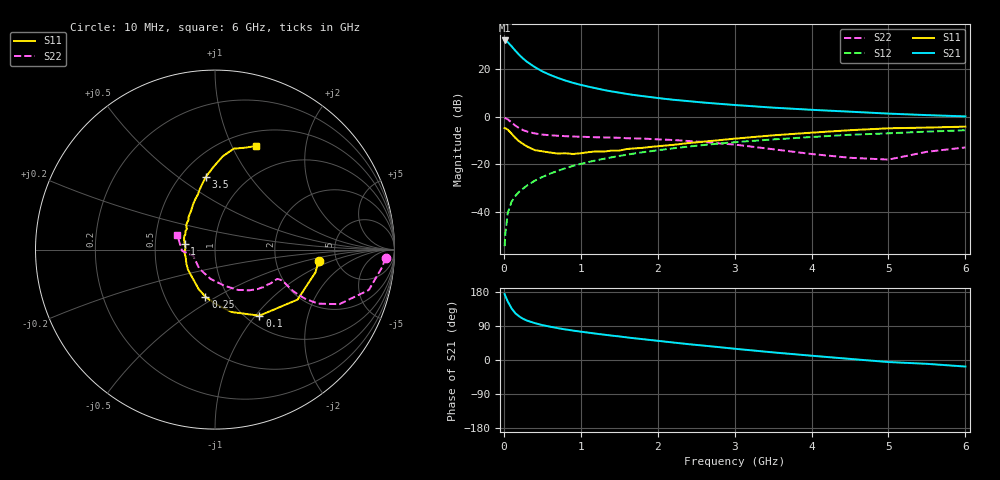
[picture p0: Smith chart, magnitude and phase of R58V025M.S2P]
! SIEMENS Small Signal Semiconductors
! BFR183
! Si NPN RF Bipolar Junction Transistor in SOT23
! VCE = 8 V  IC = 25 mA
! Common Emitter S-Parameters:  May  1996
# GHz  S  MA  R  50
!  f  S11  S21  S12  S22
! GHz  MAG  ANG  MAG  ANG  MAG  ANG  MAG  ANG
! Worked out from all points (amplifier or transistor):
!   36 points, 10 MHz to 6 GHz, reference 50 ohm
!   highest |S21| = 32.1 dB at 10 MHz (marker M1)
!   |S21| within 3 dB of that: start of sweep to 115.2 MHz
!   unconditionally stable (mu >= 1): 566.5 MHz to 2.507 GHz
!   at 250 MHz: K = 0.82, MSG = 27.4 dB, |S12| = -30.2 dB
!   at 1.4 GHz: K = 1.04, MAG = 12.6 dB, |S12| = -17.1 dB
!   at 6 GHz: K = 0.90, MSG = 2.9 dB, |S12| = -5.7 dB
!   S11 on the Smith chart (normalised r, x): 10 MHz: 3.62, -0.71; 100 MHz: 1.14, -1.05; 250 MHz: 0.79, -0.45; 1 GHz: 0.71, +0.05; 3.5 GHz: 0.66, +0.64; 6 GHz: 0.66, +1.24
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0.01  0.5804 -6.4  40.29 173.9  0.0019 83.8  0.9513 -2.8
0.02  0.5739 -12.7  39.63 168.8  0.0035 82.6  0.9357 -6.1
0.05  0.5378 -31.2  37.2 154.8  0.0094 78.8  0.8862 -14.7
0.1  0.4436 -56.1  30.51 136.4  0.0163 71.5  0.7566 -23.7
0.15  0.3594 -75.3  24.48 123.3  0.0216 69.0  0.6499 -27.6
0.2  0.3036 -89.1  20.09 115.0  0.0266 69.0  0.5754 -28.6
0.25  0.2681 -101.6  16.77 108.7  0.0308 69.5  0.524 -28.4
0.3  0.238 -112.5  14.38 104.1  0.0358 69.6  0.4903 -27.9
0.4  0.1993 -130.1  11.16 97.5  0.0449 71.3  0.4469 -26.3
0.5  0.1877 -143.5  9.023 92.1  0.0541 72.3  0.4226 -25.1
0.6  0.1773 -154.2  7.615 88.0  0.0636 72.2  0.4087 -24.8
0.7  0.1687 -166.0  6.589 84.1  0.073 72.1  0.3991 -24.8
0.8  0.1713 -174.8  5.781 80.7  0.0829 71.2  0.3906 -24.9
1  0.1713 169.2  4.691 74.8  0.1022 70.1  0.3805 -25.9
1.1  0.1799 163.2  4.303 72.2  0.1116 69.5  0.3759 -27.1
1.3  0.1855 153.2  3.664 66.9  0.1309 67.8  0.368 -29.0
1.6  0.2099 139.9  3.021 59.6  0.1596 64.8  0.3541 -33.0
2.2  0.2567 120.9  2.283 46.2  0.2171 58.5  0.3248 -42.6
3.5  0.4075 97.3  1.557 20.1  0.334 42.1  0.2077 -75.5
4.5  0.5223 85.2  1.28 2.9  0.4184 29.7  0.1372 -129.8
5.5  0.5925 73.4  1.084 -10.1  0.4872 18.4  0.1836 -177.8
6  0.621 68.4  1.019 -17.3  0.5206 11.1  0.2269 158.4
